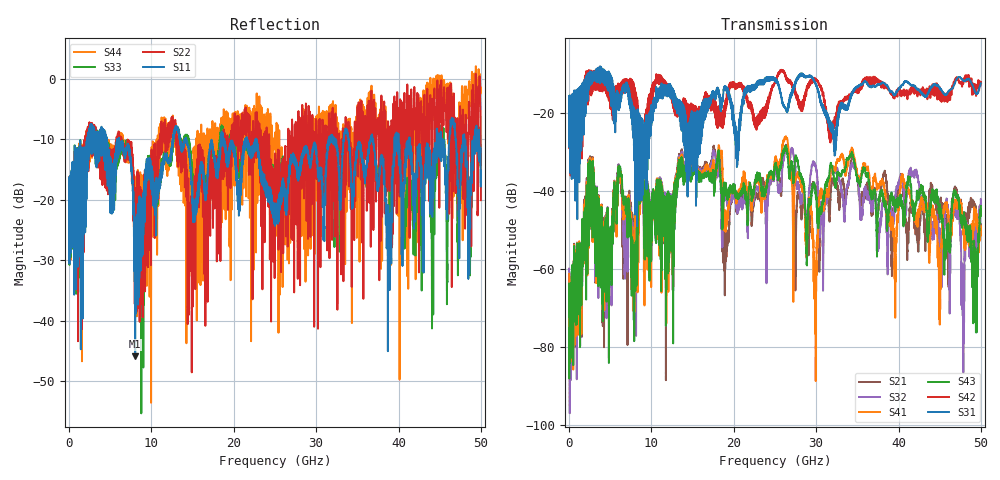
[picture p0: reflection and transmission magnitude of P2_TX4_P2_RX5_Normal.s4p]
!Keysight Technologies,N5225B,MY57041031,A.13.20.10
!Date: Friday, May 31, 2019 11:34:26
!Correction: S11(Full 4 Port(1,2,3,4))
!S12(Full 4 Port(1,2,3,4))
!S13(Full 4 Port(1,2,3,4))
!S14(Full 4 Port(1,2,3,4))
!S21(Full 4 Port(1,2,3,4))
!S22(Full 4 Port(1,2,3,4))
!S23(Full 4 Port(1,2,3,4))
!S24(Full 4 Port(1,2,3,4))
!S31(Full 4 Port(1,2,3,4))
!S32(Full 4 Port(1,2,3,4))
!S33(Full 4 Port(1,2,3,4))
!S34(Full 4 Port(1,2,3,4))
!S41(Full 4 Port(1,2,3,4))
!S42(Full 4 Port(1,2,3,4))
!S43(Full 4 Port(1,2,3,4))
!S44(Full 4 Port(1,2,3,4))
!S4P File: Measurements: <S11,S12,S13,S14>,
!<S21,S22,S23,S24>,
!<S31,S32,S33,S34>,
!<S41,S42,S43,S44>:
# Hz S  dB  R 50.0
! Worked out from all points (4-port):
!   5000 points, 10 MHz to 50 GHz, reference 50 ohm
!   strongest paths, dB at 10 MHz, 12.51 GHz, 25.01 GHz, 37.51 GHz, 50 GHz:
!     S31: -19.3, -14.3, -11.3, -12.8, -12.5
!     S42: -19.5, -17.0, -12.2, -11.8, -12.1
!     S43: -72.3, -45.9, -33.5, -45.8, -43.9
!     S41: -61.3, -45.9, -32.0, -38.8, -49.2
!     S32: -59.9, -43.9, -34.8, -55.3, -42.2
!     S21: -69.0, -44.5, -33.4, -43.7, -48.6
!   lowest |S11| = -45.9 dB at 8.03 GHz (marker M1), VSWR 1.01, Z = 50.2 - j0.466 ohm
!   |S11| at or under -10 dB: 6.073 GHz to 12.61 GHz (6.542 GHz wide, 70 % of centre); 14.21 GHz to 18.43 GHz (4.228 GHz wide, 25.9 % of centre); 22.71 GHz to 31.52 GHz (8.807 GHz wide, 32.5 % of centre)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
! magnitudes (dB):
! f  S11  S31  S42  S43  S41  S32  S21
! 10 MHz  -19.0  -19.3  -19.5  -72.3  -61.3  -59.9  -69.0
! 2.59 GHz  -11.0  -12.8  -14.9  -33.1  -32.7  -32.4  -32.0
! 8.03 GHz  -45.9  -23.3  -16.9  -58.8  -48.2  -52.8  -47.3
! 26.28 GHz  -20.1  -18.8  -10.9  -28.5  -26.2  -29.6  -29.0
! 29.9 GHz  -11.0  -12.4  -11.6  -39.4  -59.9  -33.3  -38.9
! 34.29 GHz  -17.6  -15.4  -15.2  -30.5  -29.4  -33.3  -32.0
! 50 GHz  -15.2  -12.5  -12.1  -43.9  -49.2  -42.2  -48.6
